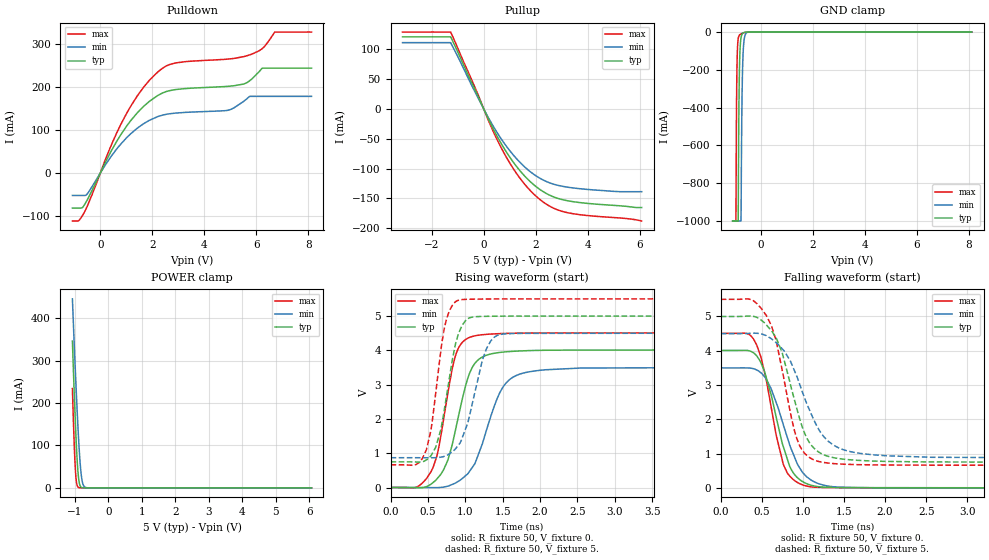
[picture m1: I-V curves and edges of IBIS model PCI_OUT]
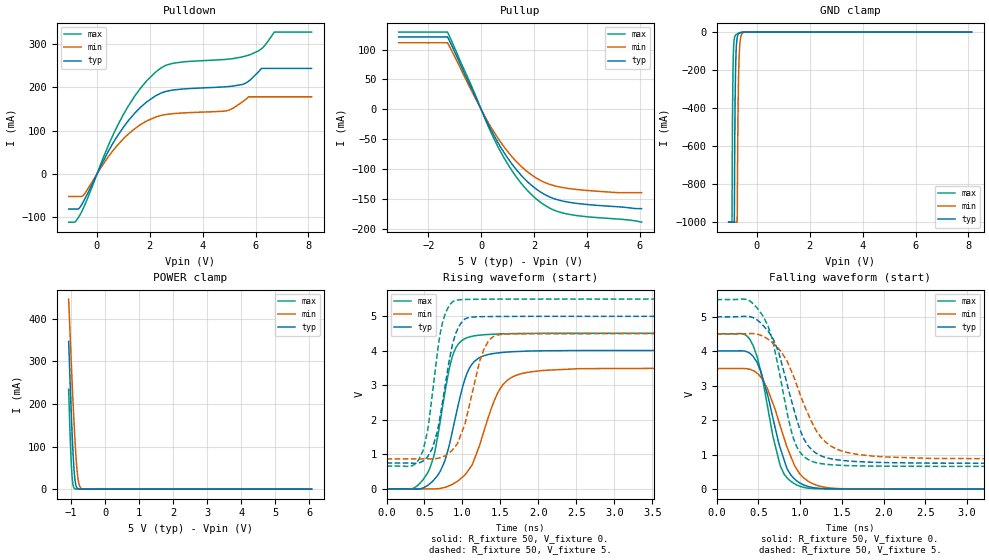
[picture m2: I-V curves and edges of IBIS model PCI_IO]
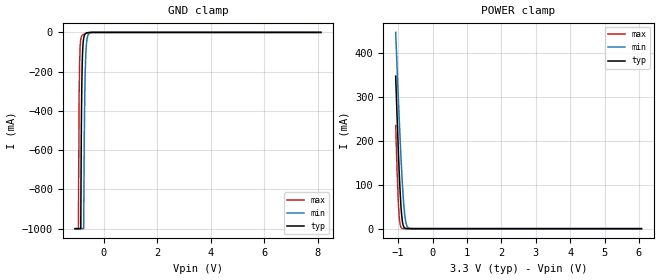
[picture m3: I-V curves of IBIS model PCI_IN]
|   IBIS Model for Tsi382 LQFP Package
[IBIS Ver]   3.2
[Disclaimer] This model is subject to change.
   Integrated Device Technology, Inc. ("IDT") hereby grants the
   user of this IBIS model a non-exclusive, nontransferable
   license to use this IBIS model under the following terms. The
   user is granted this license only to use the IBIS model and is
   not granted rights to sell, copy (except as needed to run the
   IBIS model), rent, lease or sub-license the IBIS model in
   whole or in part, or in modified form to anyone. The User may
   modify the IBIS model to suit its specific applications, but
   rights to derivative works and such modifications shall belong
   to IDT. This IBIS model is provided on an AS IS" basis and IDT
   makes absolutely no warranty with respect to the information
   contained herein. IDT DISCLAIMS AND CUSTOMER WAIVES ALL
   WARRANTIES, EXPRESS AND IMPLIED, INCLUDING WARRANTIES OF
   MERCHANTABILITY AND FITNESS FOR A PARTICULAR PURPOSE. THE
   ENTIRE RISK AS TO QUALITY AND PERFORMANCE IS WITH THE USER
   ACCORDINGLY, IN NO EVENT SHALL IDT BE LIABLE FOR ANY DIRECT OR
   INDIRECT DAMAGES, WHETHER IN CONTRACT OR TORT, INCLUDING ANY
   LOST PROFITS OR OTHER INCIDENTAL, CONSEQUENTIAL, EXEMPLARY, OR
   PUNITIVE DAMAGES ARISING OUT OF THE USE OR APPLICATION OF THE
   IBIS model. Further, IDT reserves the right to make changes
   without notice to any product herein to improve reliability,
   function, or design. IDT does not convey any license under
   patent rights or any other intellectual property rights,
   including those of third parties. IDT is not obligated to
   provide maintenance or support for the licensed IBIS model.
[Copyright]   Copyright 2009, Integrated Device Technology, Inc. all
   rights reserved.
[File Name]   tsi382_5vpci_qfp.ibs
[File Rev]   1.2
[Notes]
   Revision History
   Rev 1.0
   - 02/25/2009 Inital Release. IBIS model generated from
   SPICE model extraction. AP
   Rev 1.1
   - 08/31/2009 Updated with IDT formatting. IT
|	  Rev 1.2
   - 11/09/2009 Changed pin #136 from VDD_PCI to VIO_PCI.
[Component] Tsi382
[Manufacturer] Integrated Device Technology, Inc.
|   typ   min   max
[Package]
R_pkg   119m   116m   130m
L_pkg   7.62nH   7.61nH   8.82nH
C_pkg   0.52pF   0.46pF   0.59pF
[Pin]  signal_name   model_name   R_pin   L_pin   C_pin
6   GPIO[0]   NC   117.3m   7.7nh   0.52pf
11   GPIO[1]   NC   116.4m   7.6nh   0.52pf
9   GPIO[2]   NC   117.3m   7.7nh   0.52pf
10   GPIO[3]   NC   116.4m   7.7nh   0.53pf
97   JTAG_TCK   JTAG_IN   118.9m   7.9nh   0.54pf
98   JTAG_TDI   JTAG_IN   118.8m   7.5nh   0.54pf
86   JTAG_TDO   JTAG_OUT   132.9m   9.0nh   0.58pf
129   JTAG_TMS   JTAG_IN   128.3m   8.8nh   0.56pf
127   JTAG_TRSTn   JTAG_IN   125.0m   8.3nh   0.55pf
56   PCI_AD[0]   PCI_IO   119.0m   7.5nh   0.52pf
53   PCI_AD[1]   PCI_IO   122.1m   8.0nh   0.54pf
65   PCI_AD[10]   PCI_IO   119.3m   7.0nh   0.48pf
72   PCI_AD[11]   PCI_IO   118.1m   6.9nh   0.49pf
73   PCI_AD[12]   PCI_IO   118.6m   7.2nh   0.51pf
76   PCI_AD[13]   PCI_IO   121.1m   7.7nh   0.52pf
77   PCI_AD[14]   PCI_IO   121.2m   7.8nh   0.51pf
78   PCI_AD[15]   PCI_IO   121.0m   7.7nh   0.51pf
92   PCI_AD[16]   PCI_IO   126.0m   8.6nh   0.54pf
114   PCI_AD[17]   PCI_IO   117.8m   7.0nh   0.48pf
113   PCI_AD[18]   PCI_IO   117.6m   7.1nh   0.49pf
112   PCI_AD[19]   PCI_IO   118.8m   7.2nh   0.48pf
60   PCI_AD[2]   PCI_IO   118.4m   7.3nh   0.50pf
109   PCI_AD[20]   PCI_IO   117.0m   7.0nh   0.47pf
115   PCI_AD[21]   PCI_IO   116.8m   6.9nh   0.48pf
118   PCI_AD[22]   PCI_IO   117.4m   7.6nh   0.51pf
119   PCI_AD[23]   PCI_IO   116.6m   7.5nh   0.49pf
121   PCI_AD[24]   PCI_IO   116.3m   7.5nh   0.56pf
125   PCI_AD[25]   PCI_IO   121.1m   7.9nh   0.52pf
123   PCI_AD[26]   PCI_IO   119.7m   7.8nh   0.52pf
124   PCI_AD[27]   PCI_IO   118.9m   8.1nh   0.51pf
142   PCI_AD[28]   PCI_IO   120.1m   7.9nh   0.51pf
143   PCI_AD[29]   PCI_IO   119.6m   7.5nh   0.52pf
57   PCI_AD[3]   PCI_IO   119.3m   7.6nh   0.50pf
147   PCI_AD[30]   PCI_IO   116.8m   7.4nh   0.49pf
141   PCI_AD[31]   PCI_IO   119.7m   7.7nh   0.52pf
64   PCI_AD[4]   PCI_IO   119.3m   7.0nh   0.48pf
62   PCI_AD[5]   PCI_IO   118.0m   7.3nh   0.49pf
61   PCI_AD[6]   PCI_IO   117.5m   7.3nh   0.50pf
52   PCI_AD[7]   PCI_IO   122.3m   8.1nh   0.54pf
67   PCI_AD[8]   PCI_IO   121.1m   7.2nh   0.49pf
70   PCI_AD[9]   PCI_IO   119.2m   7.0nh   0.50pf
66   PCI_CBEn[0]   PCI_IO   121.0m   7.3nh   0.48pf
79   PCI_CBEn[1]   PCI_IO   122.2m   7.9nh   0.53pf
103   PCI_CBEn[2]   PCI_IO   114.7m   7.3nh   0.48pf
120   PCI_CBEn[3]   PCI_IO   115.7m   7.5nh   0.50pf
167   PCI_CLK   PCI_IN   122.5m   7.7nh   0.52pf
146   PCI_CLKO[0]   PCI_OUT   121.0m   7.3nh   0.50pf
51   PCI_CLKO[1]   PCI_OUT   124.8m   8.3nh   0.55pf
134   PCI_CLKO[2]   PCI_OUT   130.2m   8.9nh   0.57pf
137   PCI_CLKO[3]   PCI_OUT   123.0m   8.3nh   0.55pf
170   PCI_CLKO[4]   PCI_OUT   122.7m   7.8nh   0.54pf
96   PCI_DEVSELn   PCI_IO   120.0m   7.7nh   0.54pf
106   PCI_FRAMEn   PCI_IO   116.6m   7.2nh   0.46pf
152   PCI_GNTn[0]   PCI_IO   117.9m   6.8nh   0.76pf
155   PCI_GNTn[1]   PCI_OUT   118.8m   7.0nh   0.46pf
157   PCI_GNTn[2]   PCI_OUT   118.6m   6.9nh   0.60pf
163   PCI_GNTn[3]   PCI_OUT   118.4m   7.6nh   0.82pf
162   PCI_INTAn   PCI_IN   117.8m   7.5nh   0.54pf
161   PCI_INTBn   PCI_IN   118.1m   7.0nh   0.84pf
168   PCI_INTCn   PCI_IN   123.2m   7.9nh   0.75pf
164   PCI_INTDn   PCI_IN   119.1m   7.4nh   0.59pf
105   PCI_IRDYn   PCI_IO   115.7m   7.0nh   0.58pf
94   PCI_LOCKn   PCI_OUT   123.1m   8.2nh   0.48pf
169   PCI_M66EN   PCI_IN   124.3m   8.1nh   0.71pf
82   PCI_PAR   PCI_IO   128.8m   8.1nh   0.52pf
85   PCI_PERRn   PCI_IO   131.1m   8.7nh   0.84pf
149   PCI_PMEn   PCI_IN   119.0m   7.0nh   0.48pf
153   PCI_REQn[0]   PCI_IO   117.6m   6.9nh   0.62pf
138   PCI_REQn[1]   PCI_IN   121.8m   8.3nh   0.82pf
154   PCI_REQn[2]   PCI_IN   118.5m   6.9nh   0.52pf
148   PCI_REQn[3]   PCI_IN   119.0m   7.0nh   0.58pf
158   PCI_RSTn   PCI_OUT   118.6m   6.9nh   0.47pf
83   PCI_SERRn   PCI_IO   130.0m   8.6nh   0.48pf
102   PCI_STOPn   PCI_IO   114.1m   7.4nh   0.92pf
104   PCI_TRDYn   PCI_IO   115.4m   7.4nh   0.53pf
174   PCIE_PERSTn   NC   133.3m   8.8nh   0.70pf
22   PCIE_REFCLK_n   NC   111.3m   6.6nh   0.40pf
21   PCIE_REFCLK_p   NC   111.7m   6.6nh   0.39pf
24   PCIE_REXT   NC   111.3m   6.8nh   0.75pf
26   PCIE_RXD_n   NC   108.5m   6.6nh   0.45pf
27   PCIE_RXD_p   NC   107.0m   6.6nh   0.41pf
30   PCIE_TXD_n   NC   105.5m   7.0nh   0.41pf
29   PCIE_TXD_p   NC   105.7m   6.9nh   0.39pf
140   PWRUP_EN_ARB   GEN33_IN   119.7m   7.7nh   0.52pf
93   PWRUP_PLL_BYPASS   GEN33_IN   126.0m   8.6nh   0.54pf
48   SR_CLK   NC   132.9m   8.7nh   0.54pf
38   SR_CSn   NC   110.9m   7.5nh   0.51pf
37   SR_DIN   NC   111.8m   7.5nh   0.51pf
47   SR_DOUT   NC   132.9m   8.7nh   0.54pf
15   TEST_BCE   NC   117.0m   7.0nh   0.46pf
49   TEST_BIDR_CTL   NC   130.1m   8.6nh   0.55pf
35   TEST_ON   NC   107.2m   7.2nh   0.57pf
128   TEST_SPARE[0]   NC   126.7m   8.5nh   0.57pf
12   TEST_SPARE[1]   NC   116.8m   7.4nh   0.51pf
84   TEST_SPARE[2]   NC   130.0m   8.8nh   0.56pf
7   VDD   POWER
36   VDD   POWER
58   VDD   POWER
74   VDD   POWER
108   VDD   POWER
130   VDD   POWER
144   VDD   POWER
159   VDD   POWER
54   VDD_PCI   POWER
68   VDD_PCI   POWER
80   VDD_PCI   POWER
100   VDD_PCI   POWER
116   VDD_PCI   POWER
150   VDD_PCI   POWER
166   VDD_PCI   POWER
172   VDD_PCI   POWER
18   VDD_PCIE   POWER
33   VDD_PCIE   POWER
19   VDDA_PCIE   POWER
32   VDDA_PCIE   POWER
14   VDDA_PLL   POWER
71   VIO_PCI   POWER
111   VIO_PCI   POWER
136   VIO_PCI   POWER
173   VIO_PCI   POWER
1   VSS   GND
2   VSS   GND
3   VSS   GND
4   VSS   GND
5   VSS   GND
8   VSS   GND
13   VSS   GND
17   VSS   GND
20   VSS   GND
23   VSS   GND
25   VSS   GND
28   VSS   GND
31   VSS   GND
34   VSS   GND
39   VSS   GND
40   VSS   GND
41   VSS   GND
42   VSS   GND
43   VSS   GND
44   VSS   GND
45   VSS   GND
46   VSS   GND
50   VSS   GND
55   VSS   GND
59   VSS   GND
63   VSS   GND
69   VSS   GND
75   VSS   GND
81   VSS   GND
87   VSS   GND
88   VSS   GND
89   VSS   GND
90   VSS   GND
91   VSS   GND
95   VSS   GND
99   VSS   GND
101   VSS   GND
107   VSS   GND
110   VSS   GND
117   VSS   GND
122   VSS   GND
126   VSS   GND
131   VSS   GND
132   VSS   GND
133   VSS   GND
135   VSS   GND
139   VSS   GND
145   VSS   GND
151   VSS   GND
156   VSS   GND
160   VSS   GND
165   VSS   GND
171   VSS   GND
175   VSS   GND
176   VSS   GND
16   VSSA_PLL   GND
| Models and submodels in the file (6): PCI_OUT (Output), PCI_IO (I/O), PCI_IN (Input), JTAG_IN (Input), JTAG_OUT (Output), GEN33_IN (Input)
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[Model]   PCI_OUT
Model_type  Output
C_comp 4.536p 4.202p 4.874p
Polarity   Non-Inverting
Enable   Active-High
Vmeas =   1.32V
Cref =   10pF
Rref =   50
Vref=   0.0V
[Temperature Range]   27.0   125.0   -40.0
[Voltage Range] 5. 4.5 5.5
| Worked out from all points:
|   slope of the pulldown table from 0 to 0.75 V, typ, clamps not added: 8.81 ohm
|   slope of the pullup table from 0 to 0.75 V, typ, clamps not added: 11.8 ohm
|   GND clamp passes 1 mA (typ) near -0.58 V on its own axis
|   POWER clamp passes 1 mA (typ) near -0.80 V on its own axis
|   rising waveform, R_fixture 50, V_fixture 0.: 20-80 % time 271ps typ, 341ps min, 223ps max; typ from 0 V to 4.01 V
|   rising waveform, R_fixture 50, V_fixture 5.: 20-80 % time 204ps typ, 254ps min, 174ps max; typ from 0.748 V to 5 V
|   falling waveform, R_fixture 50, V_fixture 0.: 20-80 % time 260ps typ, 305ps min, 229ps max; typ from 4.01 V to 0 V
|   falling waveform, R_fixture 50, V_fixture 5.: 20-80 % time 307ps typ, 393ps min, 259ps max; typ from 5 V to 0.748 V
[Pulldown]
-1.072V   -80.93mA   -51.78mA   -111mA
-830.1mV  -80.93mA   -51.78mA   -110.2mA
-625.6mV  -75.05mA   -51.78mA   -92.1mA
425mV     51.67mA    39.35mA    65.16mA
1.011V    108.6mA    81.72mA    138.1mA
2.21V     179.7mA    130.8mA    234.1mA
2.879V    193.3mA    138.9mA    254.9mA
4.887V    200.8mA    145.2mA    263.9mA
5.761V    214.7mA    177.7mA    274.1mA
6.226V    243mA      177.7mA    288.2mA
6.71V     243mA      177.7mA    326.7mA
8.123V    243mA      177.7mA    326.7mA
[Pullup]
-3.123V   121mA      111.2mA    129.1mA
-1.273V   121mA      111.2mA    129.1mA
-408.1mV  39.21mA    34.71mA    43.33mA
103.2mV   -9.96mA    -8.61mA    -11.21mA
754mV     -64.09mA   -55.48mA   -71.94mA
1.433V    -105.7mA   -91.4mA    -118.6mA
1.786V    -121.9mA   -105.2mA   -136.8mA
2.186V    -135.9mA   -116.9mA   -152.8mA
2.725V    -148.2mA   -126.7mA   -167.3mA
3.264V    -154.4mA   -131.5mA   -174.5mA
4.984V    -161.7mA   -138.3mA   -182.2mA
6.072V    -165.4mA   -138.8mA   -188mA
[GND Clamp]
-1.072V   -1A        -1A        -1A
-946.2mV  -1A        -1A        -1A
-927.6mV  -1A        -1A        -477.7mA
-913.6mV  -1A        -1A        -259.6mA
-857.8mV  -1A        -1A        -35.04mA
-829.9mV  -387.1mA   -1A        -20.17mA
-792.7mV  -109.1mA   -1A        -13.52mA
-750.8mV  -31.16mA   -1A        -10.02mA
-718.2mV  -13.49mA   -425.6mA   -7.927mA
-681mV    -5.936mA   -150.7mA   -5.835mA
-541.4mV  -487.9uA   -4.567mA   -875.4uA
8.123V    0A         0A         0A
[Power Clamp]
-1.072V   346.3mA    445.7mA    234.2mA
-1.025V   239mA      352.7mA    117.5mA
-985.9mV  158.9mA    279.6mA    47.19mA
-953.7mV  100.9mA    221.8mA    15.32mA
-930mV    65.56mA    181.6mA    5.554mA
-906.4mV  38.32mA    144mA      1.868mA
-865.6mV  11.54mA    86.96mA    261.8uA
-839.8mV  4.741mA    57.78mA    114.1uA
-809.7mV  1.564mA    32.24mA    114.1uA
-764.6mV  288.3uA    10.74mA    114.1uA
-708.7mV  34.28uA    2.193mA    114.1uA
6.072V    0A         0A         0A
[Ramp]
dV/dt_r 2.406/269.779p 2.1/340.819p 2.705/222.777p
dV/dt_f 2.551/306.834p 2.179/393.351p 2.904/258.7p
[Rising Waveform]
R_fixture = 50
V_fixture = 0.
0s        0V         0V         0V
340ps     -4.676mV   86.06uV    4.549mV
540ps     94.69mV    -2.304mV   456.9mV
640ps     301mV      -2.262mV   1.113V
770ps     822.3mV    41.22mV    2.797V
860ps     1.592V     120.4mV    3.781V
1.06ns    3.349V     481.1mV    4.379V
1.46ns    3.937V     2.758V     4.487V
1.71ns    3.979V     3.291V     4.5V
4.91ns    4.01V      3.5V       4.508V
[Rising Waveform]
R_fixture = 50
V_fixture = 5.
V_fixture_min = 4.5
V_fixture_max = 5.5
0s        748.2mV    868.5mV    660.9mV
340ps     743.4mV    868.5mV    668.5mV
480ps     805.4mV    867.5mV    1.103V
610ps     1.216V     870.6mV    2.858V
720ps     2.281V     911.3mV    4.647V
890ps     4.347V     1.186V     5.445V
1.03ns    4.918V     1.86V      5.488V
1.28ns    4.991V     4.027V     5.496V
1.43ns    4.995V     4.436V     5.498V
4.91ns    5V         4.5V       5.5V
[Falling Waveform]
R_fixture = 50
V_fixture = 0.
0s        4.01V      3.5V       4.508V
400ps     3.94V      3.477V     4.342V
530ps     3.418V     3.25V      3.403V
670ps     2.118V     2.522V     1.6V
760ps     1.216V     1.855V     703.3mV
860ps     527.8mV    1.121V     291.2mV
990ps     192.2mV    470.5mV    92.32mV
1.17ns    40.8mV     141mV      16.71mV
1.44ns    9.292mV    19.45mV    6.614mV
4.91ns    8.688uV    23.08uV    4.321uV
[Falling Waveform]
R_fixture = 50
V_fixture = 5.
V_fixture_min = 4.5
V_fixture_max = 5.5
0s        5V         4.5V       5.5V
370ps     5.012V     4.511V     5.491V
560ps     4.742V     4.432V     5.006V
670ps     4.387V     4.245V     4.331V
740ps     3.99V      4.079V     3.529V
920ps     2.368V     3.287V     1.483V
1.14ns    1.146V     1.95V      809.5mV
1.37ns    882.2mV    1.249V     708.4mV
1.71ns    797.4mV    1.002V     675.1mV
4.91ns    748.3mV    869.1mV    660.9mV
[Model]   PCI_IO
Model_type  I/O
C_comp 4.536p 4.202p 4.874p
Polarity   Non-Inverting
Enable   Active-High
Vinl =   0.80V
Vinh =   2.00V
Vmeas =   1.32V
Cref =   10pF
Rref =   50
Vref=   0.0V
[Temperature Range]   27.0   125.0   -40.0
[Voltage Range] 5. 4.5 5.5
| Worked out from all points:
|   slope of the pulldown table from 0 to 0.75 V, typ, clamps not added: 8.81 ohm
|   slope of the pullup table from 0 to 0.75 V, typ, clamps not added: 11.8 ohm
|   GND clamp passes 1 mA (typ) near -0.58 V on its own axis
|   POWER clamp passes 1 mA (typ) near -0.80 V on its own axis
|   rising waveform, R_fixture 50, V_fixture 0.: 20-80 % time 271ps typ, 341ps min, 223ps max; typ from 0 V to 4.01 V
|   rising waveform, R_fixture 50, V_fixture 5.: 20-80 % time 204ps typ, 254ps min, 174ps max; typ from 0.748 V to 5 V
|   falling waveform, R_fixture 50, V_fixture 0.: 20-80 % time 260ps typ, 305ps min, 229ps max; typ from 4.01 V to 0 V
|   falling waveform, R_fixture 50, V_fixture 5.: 20-80 % time 307ps typ, 393ps min, 259ps max; typ from 5 V to 0.748 V
[Pulldown]
-1.072V   -80.93mA   -51.78mA   -111mA
-830.1mV  -80.93mA   -51.78mA   -110.2mA
-625.6mV  -75.05mA   -51.78mA   -92.1mA
425mV     51.67mA    39.35mA    65.16mA
1.011V    108.6mA    81.72mA    138.1mA
2.21V     179.7mA    130.8mA    234.1mA
2.879V    193.3mA    138.9mA    254.9mA
4.887V    200.8mA    145.2mA    263.9mA
5.761V    214.7mA    177.7mA    274.1mA
6.226V    243mA      177.7mA    288.2mA
6.71V     243mA      177.7mA    326.7mA
8.123V    243mA      177.7mA    326.7mA
[Pullup]
-3.123V   121mA      111.2mA    129.1mA
-1.273V   121mA      111.2mA    129.1mA
-408.1mV  39.21mA    34.71mA    43.33mA
103.2mV   -9.96mA    -8.61mA    -11.21mA
754mV     -64.09mA   -55.48mA   -71.94mA
1.433V    -105.7mA   -91.4mA    -118.6mA
1.786V    -121.9mA   -105.2mA   -136.8mA
2.186V    -135.9mA   -116.9mA   -152.8mA
2.725V    -148.2mA   -126.7mA   -167.3mA
3.264V    -154.4mA   -131.5mA   -174.5mA
4.984V    -161.7mA   -138.3mA   -182.2mA
6.072V    -165.4mA   -138.8mA   -188mA
[GND Clamp]
-1.072V   -1A        -1A        -1A
-946.2mV  -1A        -1A        -1A
-927.6mV  -1A        -1A        -477.7mA
-913.6mV  -1A        -1A        -259.6mA
-857.8mV  -1A        -1A        -35.04mA
-829.9mV  -387.1mA   -1A        -20.17mA
-792.7mV  -109.1mA   -1A        -13.52mA
-750.8mV  -31.16mA   -1A        -10.02mA
-718.2mV  -13.49mA   -425.6mA   -7.927mA
-681mV    -5.936mA   -150.7mA   -5.835mA
-541.4mV  -487.9uA   -4.567mA   -875.4uA
8.123V    0A         0A         0A
[Power Clamp]
-1.072V   346.3mA    445.7mA    234.2mA
-1.025V   239mA      352.7mA    117.5mA
-985.9mV  158.9mA    279.6mA    47.19mA
-953.7mV  100.9mA    221.8mA    15.32mA
-930mV    65.56mA    181.6mA    5.554mA
-906.4mV  38.32mA    144mA      1.868mA
-865.6mV  11.54mA    86.96mA    261.8uA
-839.8mV  4.741mA    57.78mA    114.1uA
-809.7mV  1.564mA    32.24mA    114.1uA
-764.6mV  288.3uA    10.74mA    114.1uA
-708.7mV  34.28uA    2.193mA    114.1uA
6.072V    0A         0A         0A
[Ramp]
dV/dt_r 2.406/269.779p 2.1/340.819p 2.705/222.777p
dV/dt_f 2.551/306.834p 2.179/393.351p 2.904/258.7p
[Rising Waveform]
R_fixture = 50
V_fixture = 0.
0s        0V         0V         0V
340ps     -4.676mV   86.06uV    4.549mV
540ps     94.69mV    -2.304mV   456.9mV
640ps     301mV      -2.262mV   1.113V
770ps     822.3mV    41.22mV    2.797V
860ps     1.592V     120.4mV    3.781V
1.06ns    3.349V     481.1mV    4.379V
1.46ns    3.937V     2.758V     4.487V
1.71ns    3.979V     3.291V     4.5V
4.91ns    4.01V      3.5V       4.508V
[Rising Waveform]
R_fixture = 50
V_fixture = 5.
V_fixture_min = 4.5
V_fixture_max = 5.5
0s        748.2mV    868.5mV    660.9mV
340ps     743.4mV    868.5mV    668.5mV
480ps     805.4mV    867.5mV    1.103V
610ps     1.216V     870.6mV    2.858V
720ps     2.281V     911.3mV    4.647V
890ps     4.347V     1.186V     5.445V
1.03ns    4.918V     1.86V      5.488V
1.28ns    4.991V     4.027V     5.496V
1.43ns    4.995V     4.436V     5.498V
4.91ns    5V         4.5V       5.5V
[Falling Waveform]
R_fixture = 50
V_fixture = 0.
0s        4.01V      3.5V       4.508V
400ps     3.94V      3.477V     4.342V
530ps     3.418V     3.25V      3.403V
670ps     2.118V     2.522V     1.6V
760ps     1.216V     1.855V     703.3mV
860ps     527.8mV    1.121V     291.2mV
990ps     192.2mV    470.5mV    92.32mV
1.17ns    40.8mV     141mV      16.71mV
1.44ns    9.292mV    19.45mV    6.614mV
4.91ns    8.688uV    23.08uV    4.321uV
[Falling Waveform]
R_fixture = 50
V_fixture = 5.
V_fixture_min = 4.5
V_fixture_max = 5.5
0s        5V         4.5V       5.5V
370ps     5.012V     4.511V     5.491V
560ps     4.742V     4.432V     5.006V
670ps     4.387V     4.245V     4.331V
740ps     3.99V      4.079V     3.529V
920ps     2.368V     3.287V     1.483V
1.14ns    1.146V     1.95V      809.5mV
1.37ns    882.2mV    1.249V     708.4mV
1.71ns    797.4mV    1.002V     675.1mV
4.91ns    748.3mV    869.1mV    660.9mV
|   MODEL PCI_IN
[Model]   PCI_IN
Model_type  Input
C_comp 4.536p 4.202p 4.874p
Polarity   Non-Inverting
Enable   Active-High
Vinl =   0.80V
Vinh =   2.00V
[Temperature Range]   27.0   125.0   -40.0
[POWER Clamp Reference]   3.30V   3.00V   3.60V
[GND Clamp Reference]   0.00V   0.00V   0.00V
[Voltage Range] 5. 4.5 5.5
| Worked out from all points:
|   GND clamp passes 1 mA (typ) near -0.58 V on its own axis
|   POWER clamp passes 1 mA (typ) near -0.80 V on its own axis
[GND Clamp]
-1.072V   -1A        -1A        -1A
-946.2mV  -1A        -1A        -1A
-927.6mV  -1A        -1A        -477.7mA
-913.6mV  -1A        -1A        -259.6mA
-857.8mV  -1A        -1A        -35.04mA
-829.9mV  -387.1mA   -1A        -20.17mA
-792.7mV  -109.1mA   -1A        -13.52mA
-750.8mV  -31.16mA   -1A        -10.02mA
-718.2mV  -13.49mA   -425.6mA   -7.927mA
-681mV    -5.936mA   -150.7mA   -5.835mA
-541.4mV  -487.9uA   -4.567mA   -875.4uA
8.123V    0A         0A         0A
[Power Clamp]
-1.072V   346.3mA    445.7mA    234.2mA
-1.025V   239mA      352.7mA    117.5mA
-985.9mV  158.9mA    279.6mA    47.19mA
-953.7mV  100.9mA    221.8mA    15.32mA
-930mV    65.56mA    181.6mA    5.554mA
-906.4mV  38.32mA    144mA      1.868mA
-865.6mV  11.54mA    86.96mA    261.8uA
-839.8mV  4.741mA    57.78mA    114.1uA
-809.7mV  1.564mA    32.24mA    114.1uA
-764.6mV  288.3uA    10.74mA    114.1uA
-708.7mV  34.28uA    2.193mA    114.1uA
6.072V    0A         0A         0A
